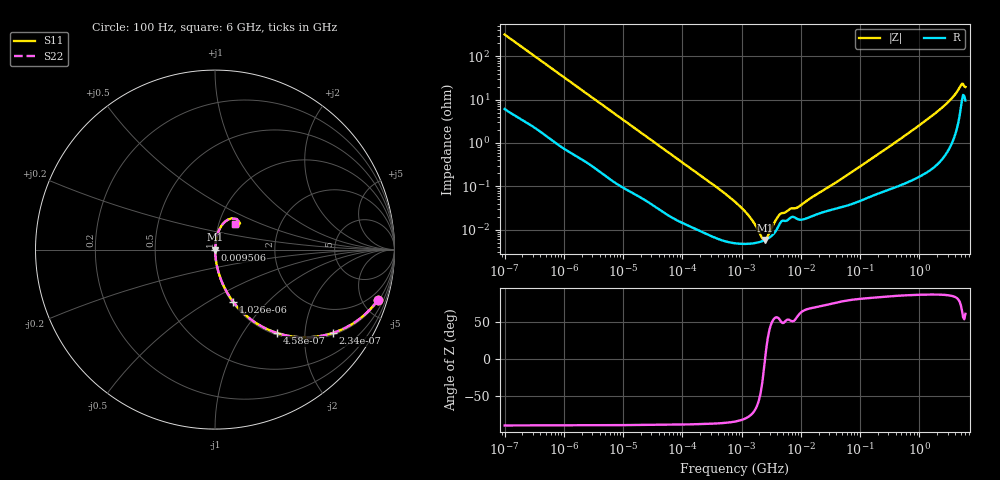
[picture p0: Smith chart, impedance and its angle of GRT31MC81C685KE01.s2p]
!Murata Part Number: GRT31MC81C685KE01
!These Parameters are Measured in Series Mode Connection
!Data Generated on Jun 19, 2026
!  o--ll--o
!Port1  Port2
!  o------o
!Operation Temp=25[degC], DC Bias Voltage=0[V]
!Freq. Start=100[Hz] Stop=6[GHz] 401[Steps]
# Hz S RI R 50
!Freq.(Hz) S11(Real) S11(Imag) S21(Real) S21(Imag) S12(Real) S12(Imag) S22(Real) S22(Imag)
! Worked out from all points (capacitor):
!   401 points, 100 Hz to 6 GHz, reference 50 ohm
!   read as one part in series: C = 4.91 uF near 109 Hz
!   lowest |Z| = 5.72 mohm at 2.481 MHz (marker M1)
!   series resonance near 2.489 MHz, so ESL is about 830 pH
!   S11 on the Smith chart (normalised r, x): 100 Hz: 1.12, -6.45; 234 Hz: 1.06, -2.78; 458 Hz: 1.03, -1.44; 1.026 kHz: 1.01, -0.65; 9.506 MHz: 1.00, +0.00; 6 GHz: 1.19, +0.35
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100  0.908 -0.2797  0.092 0.2797  0.092 0.2797  0.908 -0.2797
150  0.8195 -0.3748  0.1805 0.3748  0.1805 0.3748  0.8195 -0.3748
234  0.6566 -0.4643  0.3434 0.4643  0.3434 0.4643  0.6566 -0.4643
458  0.344 -0.4641  0.656 0.4641  0.656 0.4641  0.344 -0.4641
1026  0.1005 -0.2897  0.8995 0.2897  0.8995 0.2897  0.1005 -0.2897
2008  0.0311 -0.1615  0.9689 0.1615  0.9689 0.1615  0.0311 -0.1615
6433  0.00418 -0.053  0.9958 0.053  0.9958 0.053  0.00418 -0.053
40335  0.00037 -0.00877  0.9996 0.00877  0.9996 0.00877  0.00037 -0.00877
774597  4.84e-05 -0.000436  1 0.000436  1 0.000436  4.84e-05 -0.000436
1212075  4.68e-05 -0.000236  1 0.000236  1 0.000236  4.68e-05 -0.000236
1896632  5.05e-05 -8.38e-05  0.9999 8.38e-05  0.9999 8.38e-05  5.05e-05 -8.38e-05
2481164  5.72e-05 -1e-06  0.9999 1e-06  0.9999 1e-06  5.72e-05 -1e-06
3103719  6.88e-05 6.97e-05  0.9999 -6.97e-05  0.9999 -6.97e-05  6.88e-05 6.97e-05
4060267  0.000109 0.00016  0.9999 -0.00016  0.9999 -0.00016  0.000109 0.00016
4643984  0.000152 0.000183  0.9998 -0.000183  0.9998 -0.000183  0.000152 0.000183
9506416  0.00017 0.000304  0.9998 -0.000304  0.9998 -0.000304  0.00017 0.000304
1.555665e7  0.000205 0.000524  0.9998 -0.000524  0.9998 -0.000524  0.000205 0.000524
3.124326e8  0.00091 0.00824  0.9991 -0.00824  0.9991 -0.00824  0.00091 0.00824
2.142435e9  0.00668 0.0565  0.9933 -0.0565  0.9933 -0.0565  0.00668 0.0565
3.8344e9  0.0268 0.1172  0.9732 -0.1172  0.9732 -0.1172  0.0268 0.1172
5.016141e9  0.0934 0.1741  0.9066 -0.1741  0.9066 -0.1741  0.0934 0.1741
6e9  0.1103 0.1401  0.8897 -0.1401  0.8897 -0.1401  0.1103 0.1401
